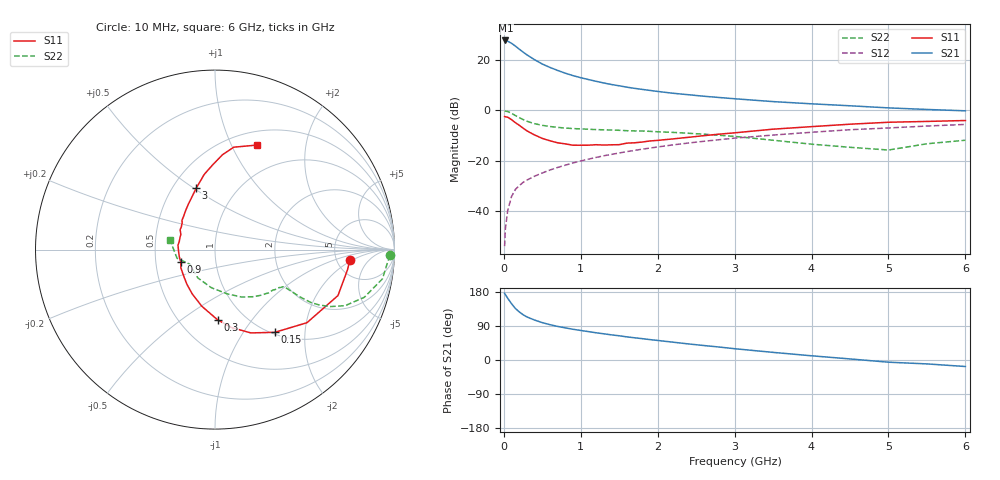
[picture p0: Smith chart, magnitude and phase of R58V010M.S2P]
! SIEMENS Small Signal Semiconductors
! BFR183
! Si NPN RF Bipolar Junction Transistor in SOT23
! VCE = 8 V  IC = 10 mA
! Common Emitter S-Parameters:  May  1996
# GHz  S  MA  R  50
!  f  S11  S21  S12  S22
! GHz  MAG  ANG  MAG  ANG  MAG  ANG  MAG  ANG
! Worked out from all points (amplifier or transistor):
!   36 points, 10 MHz to 6 GHz, reference 50 ohm
!   highest |S21| = 27.8 dB at 20 MHz (marker M1)
!   |S21| within 3 dB of that: start of sweep to 181.6 MHz
!   unconditionally stable (mu >= 1): 811.2 MHz to 2.616 GHz
!   at 250 MHz: K = 0.60, MSG = 25.9 dB, |S12| = -28.6 dB
!   at 1.4 GHz: K = 1.05, MAG = 12.5 dB, |S12| = -17.5 dB
!   at 6 GHz: K = 0.88, MSG = 2.7 dB, |S12| = -5.6 dB
!   lowest NFmin = 1.30 dB at 450 MHz
!   S11 on the Smith chart (normalised r, x): 10 MHz: 6.68, -1.71; 150 MHz: 1.03, -1.40; 300 MHz: 0.75, -0.70; 900 MHz: 0.67, -0.10; 3 GHz: 0.65, +0.51; 6 GHz: 0.65, +1.26
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0.01  0.754 -4.2  24.44 176.1  0.002 81.6  0.9766 -1.9
0.02  0.7469 -8.6  24.5 172.5  0.0044 85.8  0.9651 -4.0
0.05  0.7314 -20.5  23.66 163.0  0.0102 79.0  0.9471 -9.9
0.1  0.6544 -38.5  21.5 148.6  0.0194 73.3  0.8735 -17.7
0.15  0.569 -54.1  18.96 135.9  0.0268 67.5  0.7897 -23.3
0.2  0.5054 -66.7  16.47 127.0  0.0319 64.5  0.7166 -26.3
0.25  0.4441 -78.0  14.39 119.5  0.037 63.4  0.6571 -28.0
0.3  0.3914 -87.9  12.7 113.6  0.0411 63.2  0.6085 -28.9
0.4  0.3241 -103.1  10.14 105.4  0.0493 63.1  0.5435 -29.1
0.5  0.2773 -117.3  8.332 98.6  0.0569 63.9  0.5037 -28.8
0.6  0.2485 -129.1  7.126 93.2  0.0653 64.3  0.4774 -28.6
0.7  0.2265 -141.1  6.209 88.6  0.0734 65.1  0.459 -28.4
0.9  0.2029 -160.0  4.896 81.1  0.0902 65.2  0.4344 -28.5
1.1  0.2032 -177.4  4.093 74.9  0.1073 65.1  0.4215 -30.1
1.3  0.2042 167.0  3.497 69.1  0.1252 64.4  0.4103 -31.5
1.6  0.2233 150.5  2.888 61.0  0.1516 62.7  0.3941 -34.9
2.2  0.271 127.3  2.187 47.0  0.2062 57.9  0.3649 -43.9
3  0.3577 107.0  1.701 29.8  0.2804 49.6  0.304 -60.5
3.5  0.423 98.2  1.493 20.1  0.3229 43.5  0.2547 -75.0
4.5  0.5308 85.4  1.233 2.8  0.4124 31.6  0.1844 -121.3
5.5  0.6026 73.2  1.042 -10.3  0.4883 20.1  0.2169 -167.2
6  0.6285 68.0  0.979 -17.2  0.5255 12.6  0.2549 168.4
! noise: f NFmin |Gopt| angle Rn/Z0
0.45  1.3  0.15  45  0.18
0.9  1.4  0.2  125  0.19
1.8  2.1  0.34  -170  0.14
